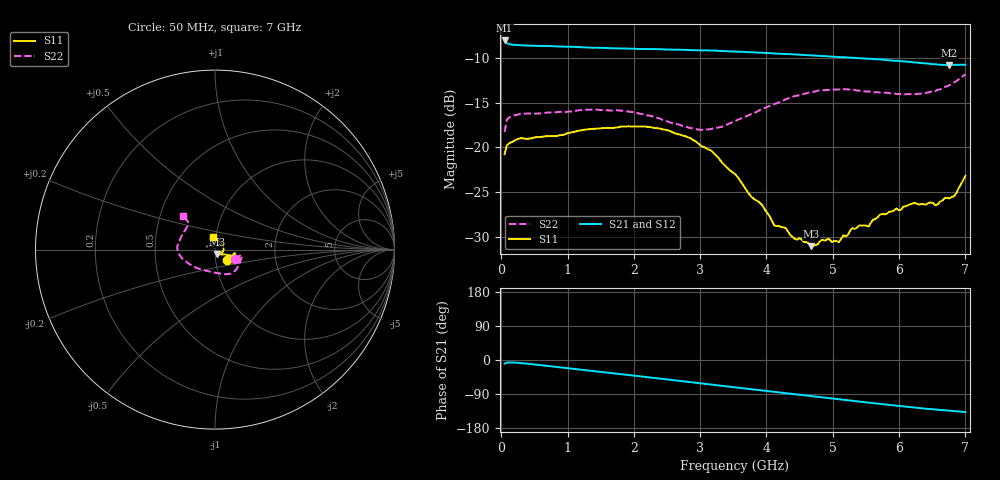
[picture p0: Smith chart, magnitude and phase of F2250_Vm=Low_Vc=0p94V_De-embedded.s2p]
! Integrated Device Technology
! Corporate Headquarters
! 6024 Silver Creek Valley Road
! San Jose, CA 95138  USA
! Phone:  1-408-284-8200
! Toll Free:  1-800-223-1366
! Webpage:  http://www.idt.com/
! Timing and RF Division
! 515 Groton Road, Suite 102
! Westford, MA 01886-6024
! Device:  F2250
! Description: Voltage Variable RF Attenuator
! Frequency:  50.0 -  6000.00 MHz
! Package:  3x3 mm Thin QFN Plastic Package: 16 pin
! Ports:  2 RF, 3 DC
!  Pin  1  = GND
!  Pin  2  = NC
!  Pin  3  = RF1  = Port 1
!  Pin  4  = NC
!  Pin  5  = GND
!  Pin  6  = GND
!  Pin  7  = GND
!  Pin  8  = GND
!  Pin  9  = NC
!  Pin 10  = RF2  = Port 2
!  Pin 11  = NC
!  Pin 12  = GND
!  Pin 13  = GND
!  Pin 14  = VCNTRL
!  Pin 15  = VDD
!  Pin 16  = VMODE
! Vcntrl:  0.940 Volts
! Vmode:  +0.000 Volts
! Vdd:  +3.30  Volts
! Current:  1.181 mA
! Data:  The device was measured on a the F2250 evaluation board which has
!  individual transmission lines to the RF pins.  Data was collected
!  using a calibrated network analyzer.  The evaluation board was
!  de-embedded using a TRL calibration technique.
!  The reference plane is the edge of the package pin.
! Misc:  SN 10
!  Action Tracker AT0258
! Date Measured:  2014-11-26
! Date:  2015-10-15  MJV
! Note:
!  Integrated Device Technology supplies this data as a sample of measured
!  data at the package pin for this product.  Your particular data for this
!  product may vary.
!  Data was taken at 25 degrees C.
!  Integrated Device Technology reserves the right to change this data at anytime.
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# GHz S dB R 50
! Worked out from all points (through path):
!   201 points, 50 MHz to 7 GHz, reference 50 ohm
!   highest |S21| = -8.06 dB at 50 MHz (marker M1); lowest = -10.8 dB at 6.757 GHz (marker M2)
!   group delay of S21, straight-line fit = 54.8 ps
!   lowest |S11| = -31.0 dB at 4.672 GHz (marker M3), VSWR 1.06, Z = 51.2 - j2.56 ohm
!   |S11| at or under -10 dB: start of sweep to end of sweep
!   |S22| runs from -18.3 to -11.8 dB; largest |S21 - S12| = 0.001
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0.05  -20.78 -41.4  -8.06 -9.5  -8.06 -9.5  -18.28 -25.6
0.08475  -19.77 -21.1  -8.37 -7.1  -8.38 -7.1  -16.89 -14.0
0.189  -19.29 -11.6  -8.55 -6.6  -8.54 -6.6  -16.45 -11.2
1.2315  -18.07 -21.8  -8.84 -26.2  -8.83 -26.2  -15.81 -42.0
2.37825  -17.88 -21.4  -9.04 -48.7  -9.03 -48.7  -16.75 -70.0
3.0385  -19.92 -20.2  -9.19 -62.1  -9.17 -62.2  -18.05 -101.6
3.525  -22.98 -25.0  -9.30 -72.2  -9.28 -72.2  -17.06 -130.8
3.76825  -25.48 -30.6  -9.39 -77.1  -9.38 -77.1  -16.28 -142.8
3.942  -26.54 -35.3  -9.44 -80.7  -9.44 -80.7  -15.71 -150.6
4.11575  -28.70 -43.0  -9.52 -84.2  -9.52 -84.2  -15.19 -157.5
4.67175  -31.04 -62.9  -9.74 -95.4  -9.73 -95.4  -13.83 -173.1
4.7065  -31.01 -65.0  -9.75 -96.1  -9.74 -96.1  -13.81 -173.8
4.915  -30.25 -63.7  -9.83 -100.3  -9.84 -100.3  -13.59 -178.4
5.08875  -30.60 -57.8  -9.92 -103.7  -9.91 -103.7  -13.55 177.6
5.29725  -29.02 -48.0  -9.99 -107.8  -9.99 -107.8  -13.56 173.1
5.5405  -28.85 -35.8  -10.11 -112.5  -10.09 -112.6  -13.75 166.7
5.85325  -27.20 -20.3  -10.27 -118.5  -10.27 -118.5  -13.95 158.5
6.33975  -26.32 15.3  -10.60 -127.4  -10.59 -127.5  -13.99 142.5
6.54825  -26.47 36.7  -10.71 -130.8  -10.72 -130.8  -13.71 136.9
6.75675  -25.71 62.0  -10.82 -133.6  -10.80 -133.7  -13.08 133.9
6.861  -25.16 76.9  -10.79 -135.2  -10.80 -135.2  -12.62 133.7
7  -23.16 97.1  -10.77 -137.3  -10.78 -137.3  -11.84 133.6
